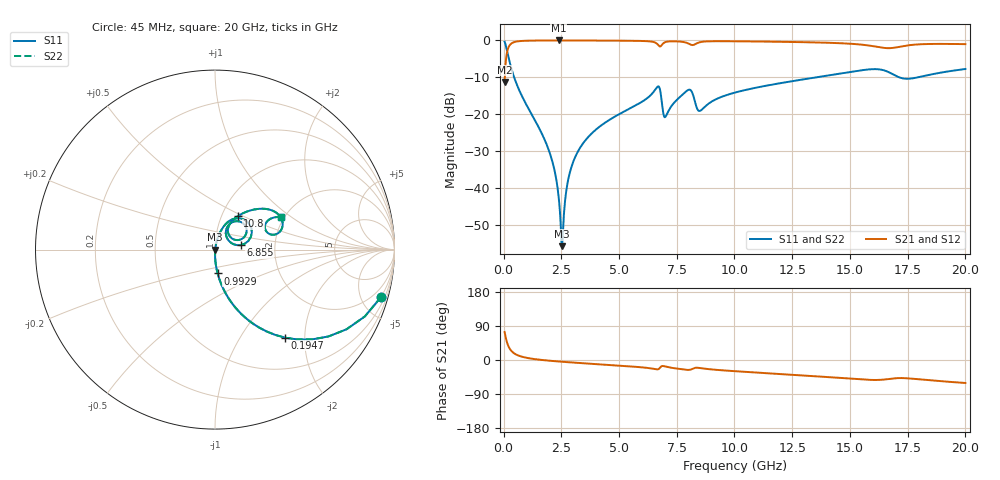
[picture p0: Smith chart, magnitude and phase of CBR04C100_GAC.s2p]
! S-parameter model data by Modelithics Inc.  support@modelithics.com 813-866-6335  Tampa FL USA
! S-Parameter data specifications:
! Substrate: 20-mil Rogers 4350B, substrate thickness, H=0.508mm, Dielectric constant, Er=3.75
! PCB Mounting Pad Footprint: Pad width, PadW=0.52mm , Pad length, PadL=0.52mm , Pad gap, PadG (edge-to-edge)=0.28mm , Reference planes=1.32mm apart
#  GHz  S  MA  R 50
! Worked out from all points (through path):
!   801 points, 45 MHz to 20 GHz, reference 50 ohm
!   highest |S21| = -0.01 dB at 2.39 GHz (marker M1); lowest = -11.2 dB at 45 MHz (marker M2)
!   group delay of S21, straight-line fit = 9.71 ps
!   lowest |S11| = -55.8 dB at 2.539 GHz (marker M3), VSWR 1.00, Z = 50.2 + j0.0357 ohm
!   |S11| at or under -10 dB: 458.1 MHz to 13.55 GHz (13.09 GHz wide, 187 % of centre); 17.13 GHz to 17.95 GHz (814.8 MHz wide, 4.65 % of centre)
!   |S22| runs from -55.8 to -0.3 dB; largest |S21 - S12| = 0
!   S11 on the Smith chart (normalised r, x): 45 MHz: 0.99, -6.98; 194.7 MHz: 0.99, -1.60; 992.9 MHz: 0.99, -0.27; 6.855 GHz: 1.33, +0.07; 10.8 GHz: 1.19, +0.46; 20 GHz: 1.92, +0.84
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0.045  0.9616 -16.0  0.2742 74.0  0.2742 74.0  0.9616 -16.0
0.194662  0.6275 -51.5  0.7783 38.5  0.7783 38.5  0.6275 -51.5
0.4441  0.3257 -71.7  0.9449 18.2  0.9449 18.2  0.3257 -71.7
0.992862  0.1335 -83.7  0.9901 5.9  0.9901 5.9  0.1335 -83.7
1.990612  0.03047 -89.3  0.9981 -1.9  0.9981 -1.9  0.03047 -89.3
2.24005  0.01545 -87.8  0.9984 -3.2  0.9984 -3.2  0.01545 -87.8
2.389712  0.007356 -82.1  0.9984 -3.9  0.9984 -3.9  0.007356 -82.1
2.464544  0.003639 -69.4  0.9984 -4.3  0.9984 -4.3  0.003639 -69.4
2.539375  0.001629 12.6  0.9984 -4.7  0.9984 -4.7  0.001629 12.6
2.863644  0.01591 77.9  0.9981 -6.1  0.9981 -6.1  0.01591 77.9
3.387462  0.03809 78.9  0.9973 -8.3  0.9973 -8.3  0.03809 78.9
6.704981  0.2385 36.4  0.8609 -24.2  0.8609 -24.2  0.2385 36.4
6.854644  0.1447 10.0  0.8678 -16.1  0.8678 -16.1  0.1447 10.0
7.02925  0.0939 45.5  0.9538 -17.6  0.9538 -17.6  0.0939 45.5
8.002056  0.2135 44.4  0.9082 -26.2  0.9082 -26.2  0.2135 44.4
8.500931  0.1108 42.2  0.9451 -21.1  0.9451 -21.1  0.1108 42.2
10.0225  0.1964 58.4  0.9731 -29.5  0.9731 -29.5  0.1964 58.4
10.79576  0.224 55.8  0.968 -32.6  0.968 -32.6  0.224 55.8
13.36496  0.3098 46.0  0.9412 -42.3  0.9412 -42.3  0.3098 46.0
16.68248  0.3711 15.1  0.7851 -50.0  0.7851 -50.0  0.3711 15.1
17.53057  0.3023 22.3  0.8585 -48.5  0.8585 -48.5  0.3023 22.3
20  0.4099 26.3  0.89 -60.7  0.89 -60.7  0.4099 26.3
